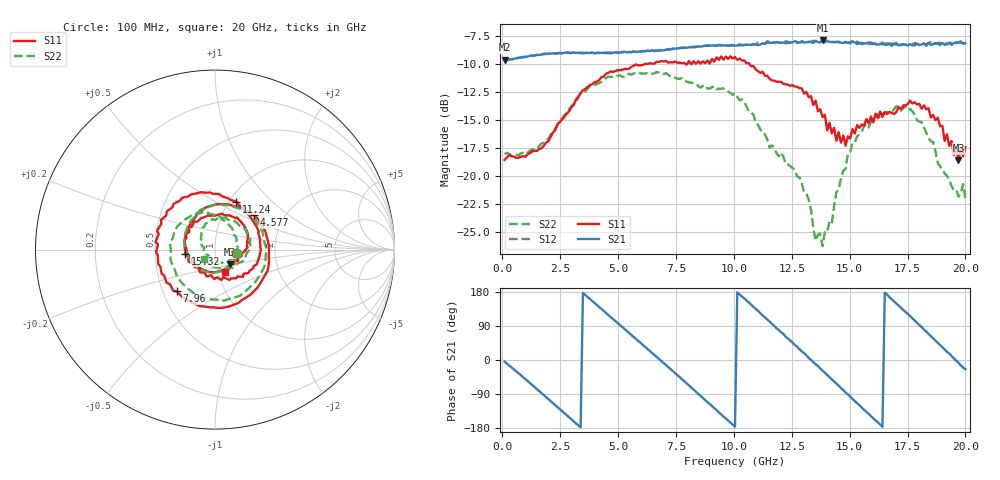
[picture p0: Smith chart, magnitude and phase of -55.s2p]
!Agilent Technologies,N5230C,MY49001569,A.09.33.09
!Agilent N5230C: A.09.33.09
!Date: Monday, July 27, 2015 20:11:01
!Correction: S11(Full 2 Port(1,2))
!S21(Full 2 Port(1,2))
!S12(Full 2 Port(1,2))
!S22(Full 2 Port(1,2))
!S2P File: Measurements: S11, S21, S12, S22:
# Hz S  dB  R 50
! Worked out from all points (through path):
!   201 points, 100 MHz to 20 GHz, reference 50 ohm
!   highest |S21| = -7.86 dB at 13.83 GHz (marker M1); lowest = -9.6 dB at 100 MHz (marker M2)
!   group delay of S21, straight-line fit = 153 ps
!   lowest |S11| = -18.6 dB at 19.7 GHz (marker M3), VSWR 1.27, Z = 58.2 - j9.75 ohm
!   |S11| at or under -10 dB: start of sweep to 6.124 GHz; 7.942295 GHz to 7.968993 GHz (26.7 MHz wide, 0.336 % of centre); 10.68 GHz to end of sweep
!   |S22| runs from -26.3 to -10.7 dB; largest |S21 - S12| = 0.014
!   S11 on the Smith chart (normalised r, x): 100 MHz: 1.26, -0.04; 4.577 GHz: 1.41, +0.59; 7.96 GHz: 0.59, -0.30; 11.24 GHz: 1.08, +0.63; 15.32 GHz: 0.71, -0.03; 20 GHz: 1.08, -0.27
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1e8  -18.57 -8.1  -9.57 -4.6  -9.59 -4.5  -18.07 -9.0
1.7915e9  -17.31 -142.0  -9.04 -92.6  -9.09 -92.3  -17.04 -139.1
2.5875e9  -14.93 157.8  -8.99 -135.2  -9.04 -135.1  -14.85 160.1
3.483e9  -12.32 100.4  -9.01 176.8  -8.95 177.0  -12.51 105.1
4.5775e9  -10.76 41.2  -9.00 118.9  -8.94 119.3  -11.10 45.0
5.672e9  -10.12 -17.0  -8.84 61.0  -8.86 61.1  -10.82 -12.3
6.7665e9  -9.78 -72.3  -8.77 2.7  -8.75 2.8  -10.75 -65.1
7.9605e9  -10.03 -132.5  -8.52 -61.8  -8.48 -61.6  -11.54 -124.5
8.9555e9  -9.93 174.8  -8.32 -116.2  -8.30 -116.1  -12.19 -179.6
1.005e10  -9.34 122.0  -8.32 -176.1  -8.29 -176.0  -12.59 122.6
1.1244e10  -10.68 66.1  -8.12 118.0  -8.10 118.3  -16.13 58.7
1.21395e10  -11.75 21.0  -8.03 68.7  -8.04 67.9  -18.28 -0.4
1.3433e10  -13.65 -40.3  -8.07 -5.6  -7.89 -4.3  -24.67 -88.6
1.3831e10  -14.72 -61.4  -7.86 -28.4  -7.88 -27.5  -26.31 -134.8
1.4826e10  -17.30 -134.5  -8.03 -85.8  -8.00 -85.0  -19.38 134.0
1.53235e10  -15.46 -172.4  -8.19 -114.1  -7.97 -113.0  -16.45 112.2
1.67165e10  -14.26 102.2  -8.11 166.2  -8.38 167.1  -14.38 47.9
1.75125e10  -13.56 56.4  -8.27 121.5  -8.31 120.3  -14.08 10.1
1.8209e10  -13.68 30.5  -8.11 80.3  -8.17 80.7  -15.68 -24.7
1.91045e10  -16.86 -11.7  -8.25 28.0  -8.02 28.5  -19.78 -77.2
1.97015e10  -18.62 -44.8  -8.02 -7.4  -8.05 -7.7  -21.87 -120.1
2e10  -17.43 -65.7  -8.10 -24.2  -8.08 -25.1  -22.03 -140.0
